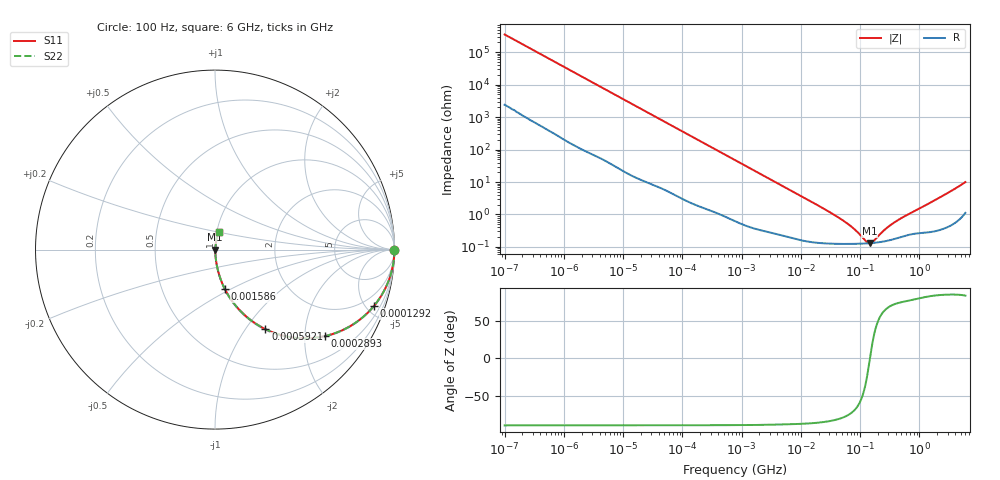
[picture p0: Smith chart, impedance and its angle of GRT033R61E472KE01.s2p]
!Murata Part Number: GRT033R61E472KE01
!These Parameters are Measured in Series Mode Connection
!Data Generated on Jun 19, 2026
!  o--ll--o
!Port1  Port2
!  o------o
!Operation Temp=25[degC], DC Bias Voltage=0[V]
!Freq. Start=100[Hz] Stop=6[GHz] 401[Steps]
# Hz S RI R 50
!Freq.(Hz) S11(Real) S11(Imag) S21(Real) S21(Imag) S12(Real) S12(Imag) S22(Real) S22(Imag)
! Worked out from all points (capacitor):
!   401 points, 100 Hz to 6 GHz, reference 50 ohm
!   read as one part in series: C = 4.49 nF near 109 Hz
!   lowest |Z| = 130 mohm at 145.9 MHz (marker M1)
!   series resonance near 147 MHz, so ESL is about 260 pH
!   S11 on the Smith chart (normalised r, x): 100 Hz: open; 129.2 kHz: 1.05, -5.63; 289.3 kHz: 1.03, -2.53; 592.1 kHz: 1.02, -1.24; 1.586 MHz: 1.01, -0.47; 6 GHz: 1.02, +0.20
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100  1 -0.000283  2e-06 0.000283  2e-06 0.000283  1 -0.000283
2008  0.9999 -0.00562  6.35e-05 0.00562  6.35e-05 0.00562  0.9999 -0.00562
12592  0.9986 -0.0349  0.00143 0.0349  0.00143 0.0349  0.9986 -0.0349
40335  0.9869 -0.1099  0.0131 0.1099  0.0131 0.1099  0.9869 -0.1099
129199  0.886 -0.3136  0.114 0.3136  0.114 0.3136  0.886 -0.3136
193316  0.7784 -0.4107  0.2216 0.4107  0.2216 0.4107  0.7784 -0.4107
289253  0.6136 -0.4816  0.3864 0.4816  0.3864 0.4816  0.6136 -0.4816
413847  0.44 -0.4906  0.56 0.4906  0.56 0.4906  0.44 -0.4906
592111  0.2804 -0.443  0.7196 0.443  0.7196 0.443  0.2804 -0.443
774597  0.1874 -0.3837  0.8126 0.3837  0.8126 0.3837  0.1874 -0.3837
1585629  0.0547 -0.2195  0.9453 0.2195  0.9453 0.2195  0.0547 -0.2195
4246196  0.00997 -0.0866  0.99 0.0866  0.99 0.0866  0.00997 -0.0866
1.555665e7  0.00197 -0.0239  0.998 0.0239  0.998 0.0239  0.00197 -0.0239
5.699437e7  0.00127 -0.00562  0.9987 0.00562  0.9987 0.00562  0.00127 -0.00562
8.154455e7  0.00125 -0.0032  0.9987 0.0032  0.9987 0.0032  0.00125 -0.0032
1.275994e8  0.00128 -0.000726  0.9987 0.000726  0.9987 0.000726  0.00128 -0.000726
1.459435e8  0.0013 -3.77e-05  0.9987 3.77e-05  0.9987 3.77e-05  0.0013 -3.77e-05
1.669249e8  0.00133 0.000648  0.9987 -0.000648  0.9987 -0.000648  0.00133 0.000648
3.124326e8  0.00161 0.00413  0.9984 -0.00413  0.9984 -0.00413  0.00161 0.00413
5.112761e8  0.00212 0.00765  0.9979 -0.00765  0.9979 -0.00765  0.00212 0.00765
2.240541e9  0.00445 0.0335  0.9955 -0.0335  0.9955 -0.0335  0.00445 0.0335
6e9  0.0205 0.0962  0.9795 -0.0962  0.9795 -0.0962  0.0205 0.0962
